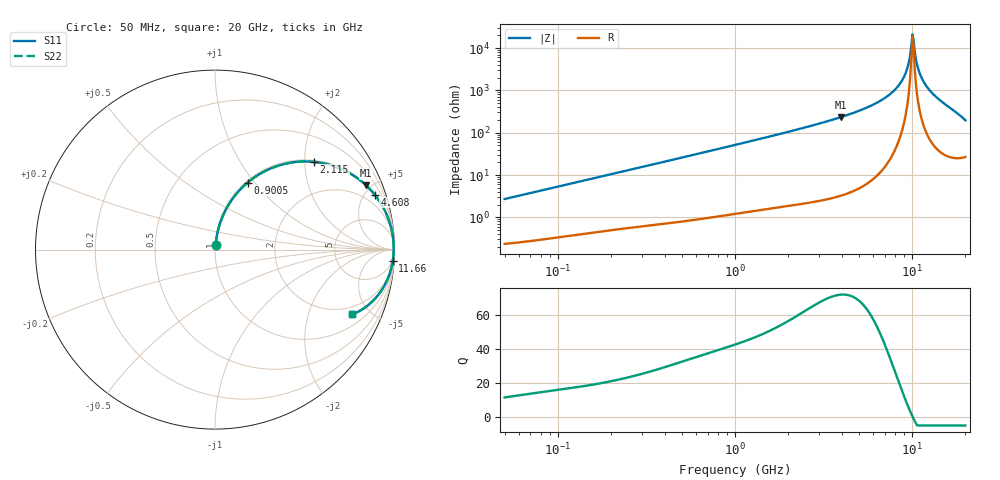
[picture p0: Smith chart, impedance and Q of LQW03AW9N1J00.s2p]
!Murata Part Number: LQW03AW9N1J00
!These Parameters are Measured in Series Mode Connection
!  o--[Z]--o
!Port1  Port2
!  o-------o
!Freq. Start=50[MHz] Stop=20[GHz], 401[Steps]
# Hz S RI R 50
!Freq.(Hz) S11(Real) S11(Imag) S21(Real) S21(Imag) S12(Real) S12(Imag) S22(Real) S22(Imag)
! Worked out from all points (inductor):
!   401 points, 50 MHz to 20 GHz, reference 50 ohm
!   read as one part in series: L = 8.55 nH near 51.52 MHz
!   highest Q = 71.8 at 3.967 GHz (marker M1), where L = 9.36 nH
!   self-resonance near 10.04 GHz
!   S11 on the Smith chart (normalised r, x): 50 MHz: 1.00, +0.05; 900.5 MHz: 1.02, +0.92; 2.115 GHz: 1.04, +2.22; 4.608 GHz: 1.08, +5.77; 11.66 GHz: 4, -31; 20 GHz: 1.53, -3.89
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5e7  0.00307 0.0268  0.9969 -0.0268  0.9969 -0.0268  0.00307 0.0268
1.364002e8  0.00909 0.071  0.9909 -0.071  0.9909 -0.071  0.00909 0.071
3.721004e8  0.0416 0.1828  0.9584 -0.1828  0.9584 -0.1828  0.0416 0.1828
9.00459e8  0.1818 0.3737  0.8182 -0.3737  0.8182 -0.3737  0.1818 0.3737
1e9  0.214 0.3985  0.786 -0.3985  0.786 -0.3985  0.214 0.3985
2.114743e9  0.552 0.4887  0.448 -0.4887  0.448 -0.4887  0.552 0.4887
2.728004e9  0.6822 0.458  0.3178 -0.458  0.3178 -0.458  0.6822 0.458
3.967106e9  0.8413 0.3585  0.1587 -0.3585  0.1587 -0.3585  0.8413 0.3585
4.608136e9  0.8892 0.3069  0.1108 -0.3069  0.1108 -0.3069  0.8892 0.3069
6.125241e9  0.9543 0.2002  0.0457 -0.2002  0.0457 -0.2002  0.9543 0.2002
7.442007e9  0.9808 0.1238  0.0192 -0.1238  0.0192 -0.1238  0.9808 0.1238
8.389408e9  0.9905 0.0759  0.0095 -0.0759  0.0095 -0.0759  0.9905 0.0759
9.041845e9  0.994 0.0454  0.00597 -0.0454  0.00597 -0.0454  0.994 0.0454
9.457416e9  0.9952 0.0269  0.0048 -0.0269  0.0048 -0.0269  0.9952 0.0269
9.892087e9  0.9956 0.00814  0.00437 -0.00814  0.00437 -0.00814  0.9956 0.00814
1.004137e10  0.9956 0.00185  0.00439 -0.00185  0.00439 -0.00185  0.9956 0.00185
1.034674e10  0.9953 -0.0108  0.00471 0.0108  0.00471 0.0108  0.9953 -0.0108
1.066139e10  0.9946 -0.0237  0.00538 0.0237  0.00538 0.0237  0.9946 -0.0237
1.098561e10  0.9936 -0.0366  0.00643 0.0366  0.00643 0.0366  0.9936 -0.0366
1.166392e10  0.9903 -0.0631  0.00974 0.0631  0.00974 0.0631  0.9903 -0.0631
1.396067e10  0.968 -0.1481  0.032 0.1481  0.032 0.1481  0.968 -0.1481
2e10  0.7646 -0.3611  0.2354 0.3611  0.2354 0.3611  0.7646 -0.3611
